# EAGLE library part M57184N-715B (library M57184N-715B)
High Voltage Input DC-to-DC Converter Source: Datasheet
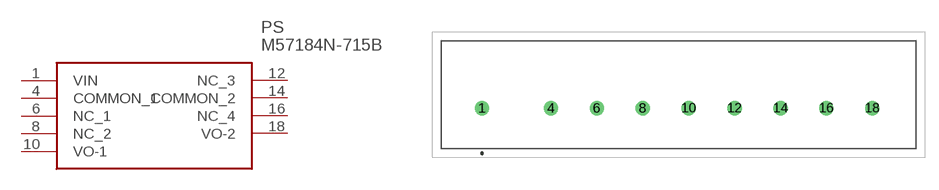
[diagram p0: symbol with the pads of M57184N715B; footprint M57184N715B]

Designator prefix PS

## M57184N-715B (Description: High Voltage Input DC-to-DC Converter; Height: 24.5mm; Manufacturer_Name: POWEREX; Manufacturer_Part_Number: M57184N-715B)  [M57184N715B]
1  VIN
4  COMMON_1
6  NC_1
8  NC_2
10  VO-1
12  NC_3
14  COMMON_2
16  NC_4
18  VO-2

## Footprint M57184N715B (pad centres in mm)
M57184N-715B-2
drill 1.05 pad 1.575: 1 0,0; 4 7.62,0; 6 12.7,0; 8 17.78,0; 10 22.86,0; 12 27.94,0; 14 33.02,0; 16 38.1,0; 18 43.18,0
